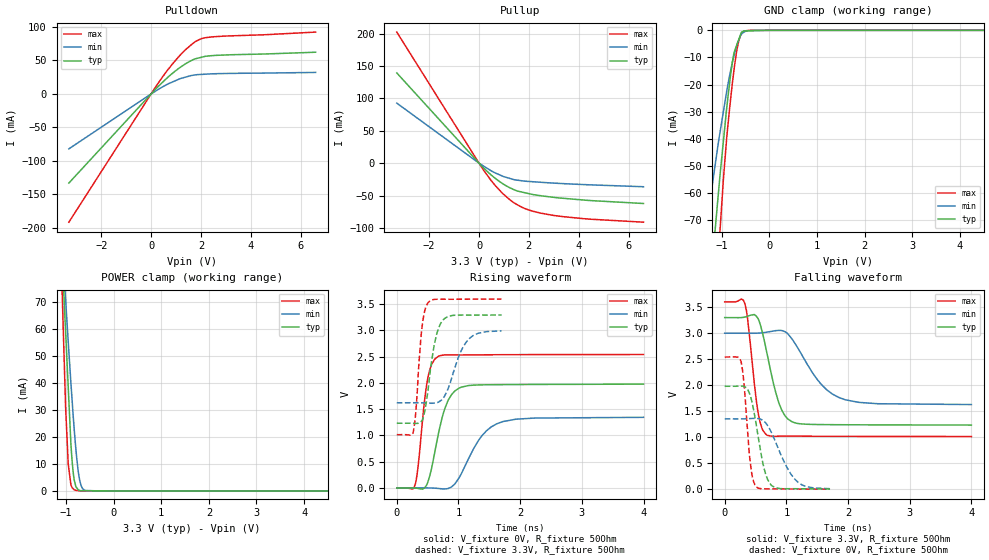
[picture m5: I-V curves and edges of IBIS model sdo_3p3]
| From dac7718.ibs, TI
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|   sdo_3p3 Model
[Model]   sdo_3p3
Model_type   3-state
Polarity   Non-Inverting
Vmeas = 1.65
Vref = 1.65
Cref = 5pF
Rref = 50
|   typ   min   max
|   (Nom PVT)   (Fast PVT)   (Slow PVT)
|C_comp from frequency method(F=50MHz)
|Average
|C_comp   3.530e-12   2.874e-12   4.123e-12
|ON state : BUFFER OUTPUT TURNED HIGH
|C_comp   4.259e-12   3.297e-12   5.137e-12
|OFF state: BUFFER IN HIGH IMPEDANCE
|C_comp   3.713e-12   2.774e-12   4.526e-12
|C_comp from LC Tank Method (L=1nH)
|Resonant Frequency(Hz)   2.68e9   2.97e9   2.48e9
C_comp   3.530e-12   2.874e-12   4.123e-12
| Where nom  PVT is Nominal Process,  3.3V,  33C
|   Fast PVT is Strong Process,   3.6V,  -40C
|   Slow PVT is Weak Process,   3V,  113C
[Voltage Range]   3.3   3   3.6
|Ambient Temperature   25   85   -40
|Junction Temperature
[Temperature Range]   33   113   -40
[Pullup Reference]   3.3   3   3.6
[Pulldown Reference]   0   0   0
[Power Clamp Reference]   3.3   3   3.6
[GND Clamp Reference]   0   0   0
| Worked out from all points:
|   slope of the pulldown table from 0 to 0.495 V, typ, clamps not added: 26.5 ohm
|   slope of the pullup table from 0 to 0.495 V, typ, clamps not added: 26.7 ohm
|   GND clamp passes 1 mA (typ) near -0.60 V on its own axis
|   POWER clamp passes 1 mA (typ) near -0.77 V on its own axis
|   falling waveform, V_fixture 3.3V, R_fixture 50Ohm: 20-80 % time 246ps typ, 485ps min, 144ps max; typ from 3.3 V to 1.24 V
|   rising waveform, V_fixture 0V, R_fixture 50Ohm: 20-80 % time 234ps typ, 399ps min, 140ps max; typ from 0 V to 1.98 V
|   rising waveform, V_fixture 3.3V, R_fixture 50Ohm: 20-80 % time 156ps typ, 259ps min, 97.1ps max; typ from 1.23 V to 3.29 V
|   falling waveform, V_fixture 0V, R_fixture 50Ohm: 20-80 % time 180ps typ, 320ps min, 103ps max; typ from 1.98 V to 0.008 V
[Pulldown]
|   Voltage   I(typ)   I(min)   I(max)
-3.3V     -132.9mA   -81.92mA   -191.3mA
378mV     14.52mA    8.811mA    21.14mA
633.6mV   23.58mA    14.06mA    34.2mA
1.17V     39.67mA    22.89mA    58.05mA
1.706V    51.44mA    28.01mA    76.28mA
2.012V    54.64mA    29.11mA    82.4mA
2.473V    57.2mA     30.04mA    85.21mA
6.6V      62.22mA    32.08mA    92.26mA
[GND Clamp]
|   Voltage   I(typ)   I(min)   I(max)
-3.3V     -567.3mA   -382.9mA   -795.5mA
-1.368V   -120.2mA   -78.23mA   -173.2mA
-1.275V   -100.6mA   -66.04mA   -144.9mA
-1.211V   -87.19mA   -58.2mA    -125.5mA
-1.071V   -59.65mA   -41.04mA   -82.86mA
-1.04V    -53.46mA   -37.64mA   -73.92mA
-896.4mV  -28.22mA   -22.21mA   -39.2mA
-811.8mV  -15.67mA   -14.52mA   -24.62mA
-734.4mV  -7.731mA   -8.474mA   -13.03mA
-651.6mV  -3.708mA   -3.831mA   -4.309mA
-537.9mV  -225.7uA   -689.5uA   -354.6uA
6.6V      0A         0A         0A
[Pullup]
|   Voltage   I(typ)   I(min)   I(max)
-3.3V     139.3mA    92.69mA    202.4mA
172.8mV   -6.962mA   -4.249mA   -10.24mA
633.6mV   -22.98mA   -14.85mA   -33.86mA
939.6mV   -31.49mA   -20.02mA   -46.56mA
1.246V    -38.25mA   -23.71mA   -56.88mA
1.554V    -43.23mA   -26.4mA    -64.58mA
1.865V    -45.92mA   -27.93mA   -70.51mA
2.473V    -50.3mA    -29.55mA   -77.2mA
2.934V    -52.53mA   -30.71mA   -80.4mA
4.316V    -57.38mA   -33.3mA    -86.12mA
6.6V      -62.36mA   -36.46mA   -91.22mA
[POWER Clamp]
|   Voltage   I(typ)   I(min)   I(max)
-3.3V     324mA      292.8mA    324.9mA
-1.282V   160.8mA    145.8mA    190.9mA
-1.012V   59.83mA    71.35mA    32.24mA
-954mV    38.29mA    55.1mA     9.849mA
-897.6mV  17.2mA     39.81mA    2.274mA
-881.1mV  13.02mA    35.63mA    1.577mA
-848.1mV  6.574mA    27.35mA    767.1uA
-810mV    2.713mA    18.71mA    269.5uA
-717mV    210.1uA    4.219mA    32.79uA
-654mV    88.94uA    886.5uA    5.267uA
-591mV    80.33uA    148uA      3.723uA
6.6V      0A         0A         0A
[Ramp]
R_load = 50
|   typ   min   max
dV/dt_r   1.18676/2.32606e-10   0.807438/3.9711e-10   1.52522/1.39476e-10
dV/dt_f   1.23903/2.45569e-10   0.822684/4.82677e-10   1.55079/1.44127e-10
[Falling Waveform]
V_fixture = 3.3V
V_fixture_min = 3V
V_fixture_max = 3.6V
R_fixture = 50Ohm
|   Time   V(typ)   V(min)   V(max)
0s        3.3V       3V         3.6V
324ps     3.309V     2.999V     3.574V
373ps     3.325V     2.999V     3.259V
540ps     3.282V     3.002V     1.486V
688ps     2.599V     3.021V     1.039V
892ps     1.615V     3.054V     1.022V
1.111ns   1.289V     2.856V     1.023V
1.562ns   1.245V     2.021V     1.019V
1.956ns   1.241V     1.72V      1.018V
3.999ns   1.235V     1.629V     1.015V
[Rising Waveform]
V_fixture = 0V
V_fixture_min = 0V
V_fixture_max = 0V
R_fixture = 50Ohm
|   Time   V(typ)   V(min)   V(max)
0s        1.527nV    2.067nV    1.282nV
300ps     -2.282mV   342uV      73.84mV
496ps     90.71mV    920.4uV    2.046V
565ps     379.5mV    -827.2uV   2.351V
675ps     1.034V     -9.36mV    2.508V
781ps     1.519V     -17.97mV   2.534V
946ps     1.851V     83.79mV    2.534V
1.376ns   1.964V     988.6mV    2.536V
1.719ns   1.968V     1.265V     2.538V
3.999ns   1.978V     1.346V     2.542V
[Rising Waveform]
V_fixture = 3.3V
V_fixture_min = 3V
V_fixture_max = 3.6V
R_fixture = 50Ohm
|   Time   V(typ)   V(min)   V(max)
0s        1.233V     1.623V     1.015V
264ps     1.231V     1.623V     1.049V
309ps     1.23V      1.623V     1.455V
404ps     1.277V     1.621V     3.01V
448ps     1.431V     1.619V     3.349V
506ps     1.858V     1.616V     3.529V
636ps     2.881V     1.622V     3.594V
764ps     3.217V     1.73V      3.596V
1.126ns   3.293V     2.78V      3.596V
1.699ns   3.295V     2.992V     3.598V
[Falling Waveform]
V_fixture = 0V
V_fixture_min = 0V
V_fixture_max = 0V
R_fixture = 50Ohm
|   Time   V(typ)   V(min)   V(max)
0s        1.98V      1.354V     2.542V
263ps     1.984V     1.354V     2.465V
315ps     1.975V     1.355V     2.001V
417ps     1.792V     1.36V      492.3mV
505ps     1.288V     1.364V     56.38mV
639ps     400.7mV    1.306V     10.57mV
763ps     70.81mV    1.079V     9.973mV
1.006ns   11.74mV    428.4mV    7.714mV
1.187ns   11.51mV    136.7mV    6.195mV
1.707ns   8.071mV    13.18mV    3.335mV
